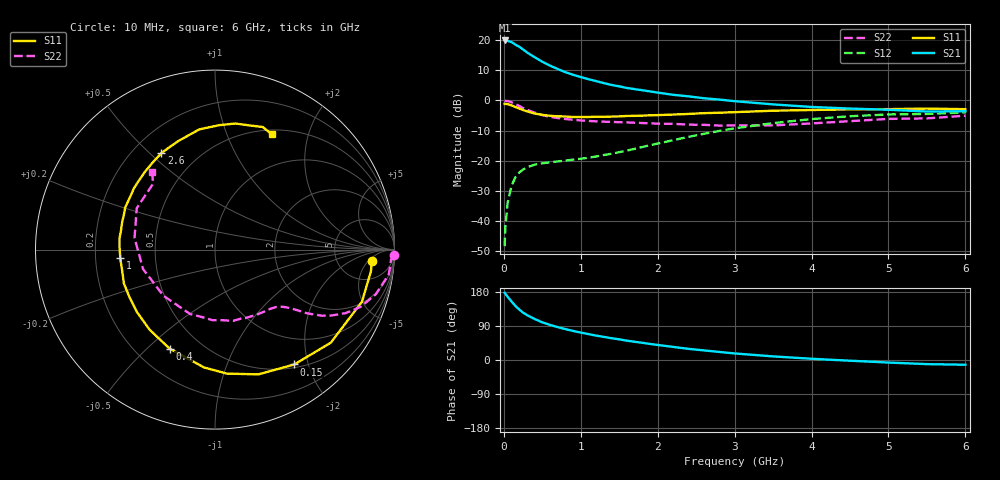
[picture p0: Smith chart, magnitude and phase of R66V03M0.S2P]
! SIEMENS Small Signal Semiconductors
! BFR193
! Si NPN RF Bipolar Junction Transistor in SOT23
! VCE = 6 V  IC = 3 mA
! Common Emitter S-Parameters:  May  1996
# GHz  S  MA  R  50
!  f  S11  S21  S12  S22
! GHz  MAG  ANG  MAG  ANG  MAG  ANG  MAG  ANG
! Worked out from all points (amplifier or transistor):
!   36 points, 10 MHz to 6 GHz, reference 50 ohm
!   highest |S21| = 19.9 dB at 10 MHz (marker M1)
!   |S21| within 3 dB of that: start of sweep to 250.1 MHz
!   unconditionally stable (mu >= 1): 1.056 GHz to 2.025 GHz
!   at 250 MHz: K = 0.30, MSG = 19.9 dB, |S12| = -23.0 dB
!   at 1.4 GHz: K = 1.09, MAG = 9.6 dB, |S12| = -17.7 dB
!   at 6 GHz: K = 0.98, MSG = 0.2 dB, |S12| = -4.0 dB
!   S11 on the Smith chart (normalised r, x): 10 MHz: 12, -6; 150 MHz: 0.55, -1.77; 400 MHz: 0.34, -0.59; 1 GHz: 0.31, -0.04; 2.6 GHz: 0.31, +0.54; 6 GHz: 0.56, +1.46
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0.01  0.8752 -4.2  9.917 177.6  0.0038 85.5  0.9952 -1.7
0.02  0.8773 -7.8  9.747 174.6  0.0079 89.1  0.9825 -3.3
0.05  0.8688 -19.5  9.743 166.8  0.0203 79.7  0.9783 -8.1
0.1  0.8278 -38.8  9.33 154.4  0.0383 69.8  0.9301 -15.5
0.15  0.7775 -55.4  8.456 142.7  0.0528 62.0  0.8725 -21.4
0.2  0.7361 -70.8  7.804 133.3  0.0634 55.9  0.8098 -25.9
0.25  0.6942 -84.5  7.022 125.0  0.0712 50.7  0.7477 -29.4
0.3  0.6595 -95.3  6.281 118.6  0.0775 47.4  0.7013 -31.7
0.4  0.6066 -114.7  5.23 108.2  0.0857 42.5  0.6264 -34.6
0.5  0.576 -129.3  4.395 99.5  0.0904 40.5  0.5692 -36.4
0.6  0.5569 -141.4  3.789 92.6  0.0938 40.0  0.5337 -37.7
0.8  0.5414 -159.7  2.945 81.5  0.1001 41.4  0.4922 -40.3
1  0.5298 -174.7  2.444 72.3  0.1075 45.4  0.4662 -43.4
1.1  0.5318 179.0  2.256 68.4  0.1119 47.8  0.457 -45.5
1.3  0.5346 168.5  1.939 61.0  0.1241 52.0  0.4437 -49.5
1.6  0.5527 154.9  1.612 51.0  0.1469 57.3  0.4316 -56.9
2.2  0.5831 132.2  1.24 34.5  0.2185 61.1  0.4097 -75.7
2.6  0.6149 119.1  1.088 25.4  0.2789 58.6  0.3935 -91.9
3.5  0.6757 97.4  0.86 9.5  0.4203 45.0  0.3854 -138.1
4.5  0.7117 80.8  0.733 -1.9  0.5472 26.0  0.4529 171.8
5.5  0.733 68.8  0.654 -10.9  0.5963 7.5  0.5037 133.2
6  0.7163 63.6  0.663 -12.5  0.6322 2.3  0.5575 129.0
